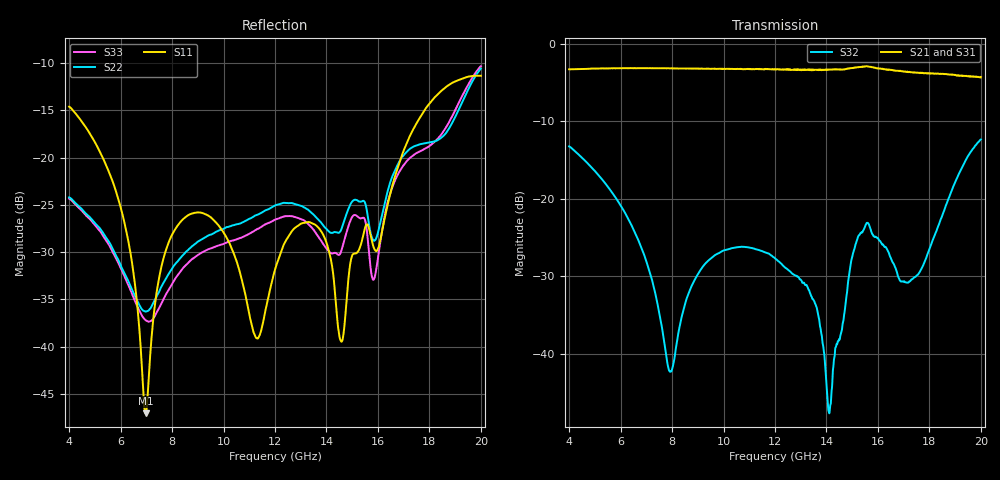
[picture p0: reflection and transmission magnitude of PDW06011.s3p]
!The following data was pulled from an Agilent PNA
!This sNp file was generated from the data in the RF Test software
!NOTE:  Smoothing/Math/Corrections applied on any given trace ARE included in the data saved here
# MHz S dB R 50
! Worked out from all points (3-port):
!   1601 points, 4 GHz to 20 GHz, reference 50 ohm
!   strongest paths, dB at 4 GHz, 8 GHz, 12 GHz, 16 GHz, 20 GHz:
!     S21: -3.3, -3.2, -3.3, -3.1, -4.3
!     S31: -3.3, -3.2, -3.3, -3.2, -4.3
!     S32: -13.2, -42.0, -27.7, -25.1, -12.3
!   lowest |S11| = -47.0 dB at 6.97 GHz (marker M1), VSWR 1.01, Z = 50.1 - j0.435 ohm
!   |S11| at or under -10 dB: start of sweep to end of sweep
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4000  -14.62 90.4  -3.29 -108.5  -3.29 -108.9
      -3.29 -108.4  -24.21 -58.7  -13.24 -139.4
      -3.30 -108.8  -13.24 -139.4  -24.33 -58.3
6050  -25.75 35.6  -3.15 -167.7  -3.15 -168.4
      -3.14 -167.7  -31.69 -122.4  -21.12 166.5
      -3.14 -168.3  -21.11 166.4  -31.93 -127.1
6970  -47.03 -77.0  -3.15 164.9  -3.16 164.2
      -3.15 164.9  -36.28 -97.8  -27.76 146.3
      -3.16 164.2  -27.76 146.3  -37.19 -108.7
7900  -28.75 175.5  -3.16 136.8  -3.17 136.1
      -3.17 136.7  -32.17 -70.4  -42.23 -169.7
      -3.16 136.0  -42.21 -169.4  -33.83 -75.0
8370  -26.67 159.7  -3.17 122.4  -3.18 121.6
      -3.18 122.4  -30.47 -70.6  -35.29 -112.7
      -3.19 121.5  -35.28 -112.7  -31.87 -74.5
12000  -31.84 -106.8  -3.28 5.1  -3.30 4.1
       -3.29 5.3  -25.07 -82.8  -27.67 170.5
       -3.29 4.3  -27.68 170.4  -26.56 -85.6
14110  -30.04 130.0  -3.31 -69.1  -3.34 -70.1
       -3.34 -69.0  -27.86 -89.5  -47.69 -176.0
       -3.38 -70.1  -47.68 -175.0  -29.96 -94.7
15250  -29.82 -132.1  -3.02 -112.9  -3.03 -114.3
       -3.01 -112.9  -24.62 -82.1  -24.76 -135.7
       -3.02 -114.1  -24.76 -135.6  -26.33 -86.8
16700  -21.65 -34.4  -3.42 -174.7  -3.43 -175.8
       -3.48 -174.9  -21.14 -65.8  -29.07 159.3
       -3.50 -176.1  -29.10 159.4  -22.20 -65.9
20000  -11.35 165.1  -4.50 39.9  -4.45 38.4
       -4.30 39.4  -10.60 32.9  -12.31 157.8
       -4.28 37.9  -12.35 158.1  -10.34 34.3
